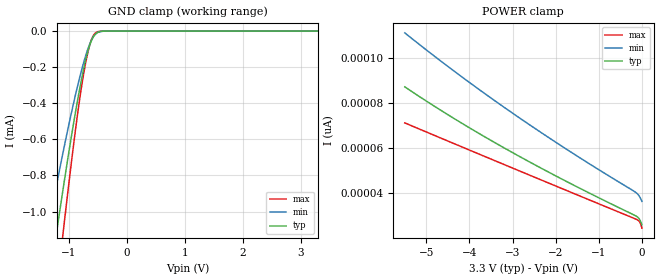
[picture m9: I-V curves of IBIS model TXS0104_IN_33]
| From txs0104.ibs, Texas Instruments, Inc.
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[Model]   TXS0104_IN_33
Model_type  Input
Vinl=0.8
Vinh=2.0
| variable   typ   min   max
C_comp   0.22pF   0.16pF   0.26pF
[Temperature Range]   40   100   -40
| Ambient temperature   25   85   -40
[Voltage range]   3.3   3   3.6
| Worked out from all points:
|   GND clamp passes 1 mA (typ) near -1.16 V on its own axis
[GND Clamp]
| TXS0104_IN_33
|   Voltage   I(typ)   I(min)   I(max)
-5.5V     -12.44mA   -9.732mA   -15.69mA
-1.395V   -1.529mA   -1.163mA   -1.988mA
-1.34V    -1.404mA   -1.069mA   -1.823mA
-1.195V   -1.082mA   -826.4uA   -1.395mA
-1.105V   -889.2uA   -681.8uA   -1.138mA
-1.08V    -836.8uA   -642.6uA   -1.068mA
-895mV    -468.8uA   -368.1uA   -573.6uA
-755mV    -226.3uA   -187.7uA   -258.9uA
-635mV    -74.55uA   -68.66uA   -73.26uA
-535mV    -15.06uA   -15.03uA   -9.098uA
-365mV    -209.3nA   -310nA     -27.85nA
3.3V      26.09pA    42.3pA     19.82pA
[POWER Clamp]
| TXS0104_IN_33
|   Voltage   I(typ)   I(min)   I(max)
-5.5V     87.15pA    111pA      71.18pA
-4.29V    72.34pA    93.17pA    61.47pA
-2.97V    57.71pA    75.1pA     50.95pA
-1.65V    44.28pA    58.31pA    40.49pA
-140mV    29.98pA    40.36pA    28.58pA
-55mV     28.47pA    38.58pA    27.43pA
-30mV     27.55pA    37.7pA     26.47pA
-95.1fV   26.09pA    36.45pA    24.57pA
